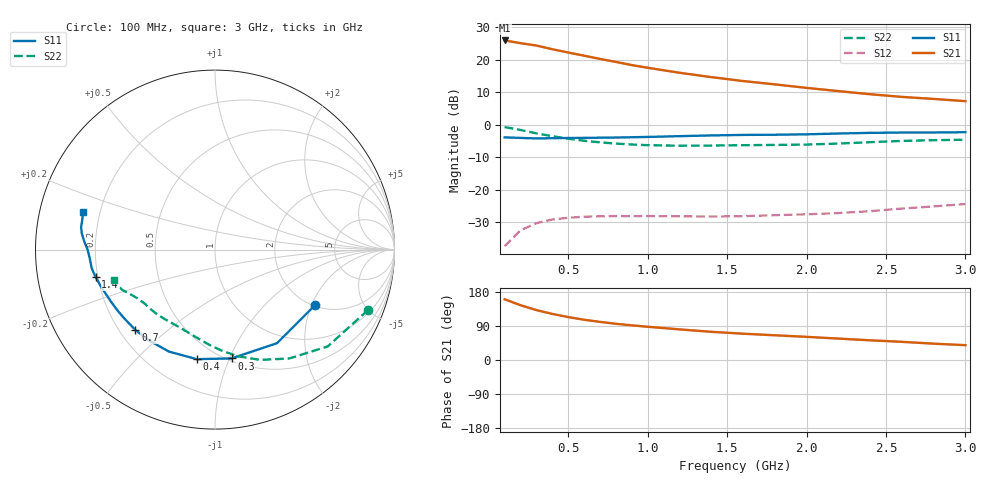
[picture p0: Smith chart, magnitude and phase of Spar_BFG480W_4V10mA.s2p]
! Filename: 410BFG480.001
! Title: BFG480W
! Bias: Vce=4V; Ic=10mA
! Company: NXP Semiconductors NL
! User: Quality&Reliability T&D
! Measure time: 10 Nov 1999 / 12:02:13
#  MHz  S  MA  R 50
! Freq  S11  S21  S12  S22  :
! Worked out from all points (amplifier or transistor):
!   20 points, 100 MHz to 3 GHz, reference 50 ohm
!   highest |S21| = 25.9 dB at 100 MHz (marker M1)
!   |S21| within 3 dB of that: start of sweep to 430.3 MHz
!   unconditionally stable (mu >= 1): 1.674 GHz to end of sweep
!   at 400 MHz: K = 0.24, MSG = 26.2 dB, |S12| = -29.2 dB
!   at 1.2 GHz: K = 0.73, MSG = 22.1 dB, |S12| = -28.2 dB
!   at 3 GHz: K = 1.15, MAG = 13.5 dB, |S12| = -24.4 dB
!   S11 on the Smith chart (normalised r, x): 100 MHz: 2.02, -2.12; 300 MHz: 0.52, -1.02; 400 MHz: 0.39, -0.77; 700 MHz: 0.26, -0.39; 1.4 GHz: 0.19, -0.11; 3 GHz: 0.14, +0.14
100  0.6371 -29.2  19.67 160.2  0.01355 67.4  0.9169 -21.5
200  0.6254 -56.5  17.86 144.6  0.02379 56.2  0.828 -40.6
300  0.6132 -81.3  16.43 131.7  0.0306 47.3  0.7346 -55.6
400  0.6188 -99.5  14.42 121.7  0.03478 40.4  0.6642 -67.7
500  0.6235 -114.3  12.84 113.3  0.03704 35.7  0.6077 -77.9
600  0.6257 -126.0  11.48 106.2  0.03838 32.5  0.5653 -85.9
700  0.6301 -134.7  10.24 100.6  0.03903 30.6  0.5345 -92.7
800  0.6335 -141.9  9.197 95.6  0.03931 29.5  0.5113 -98.5
900  0.6396 -147.4  8.227 91.5  0.03928 29.2  0.4951 -103.8
1000  0.647 -152.7  7.487 87.7  0.03935 29.4  0.4836 -108.8
1200  0.6649 -160.9  6.272 80.8  0.03904 30.9  0.4744 -117.7
1400  0.6825 -166.9  5.374 74.4  0.03864 33.7  0.4771 -125.0
1600  0.6947 -171.5  4.681 69.4  0.03917 38.1  0.4828 -130.9
1800  0.6995 -175.9  4.157 65.2  0.04062 43.4  0.4875 -136.4
2000  0.7095 -179.9  3.673 61.1  0.04183 48.4  0.494 -142.4
2200  0.7304 176.3  3.277 56.5  0.04377 52.7  0.5116 -148.2
2400  0.7475 173.1  2.934 51.9  0.04677 56.4  0.5376 -152.9
2600  0.7564 170.4  2.669 47.9  0.05132 59.8  0.5623 -156.4
2800  0.7576 167.5  2.482 43.1  0.05539 61.5  0.5766 -159.5
3000  0.7643 164.3  2.296 39.2  0.06017 63.4  0.5861 -163.4
